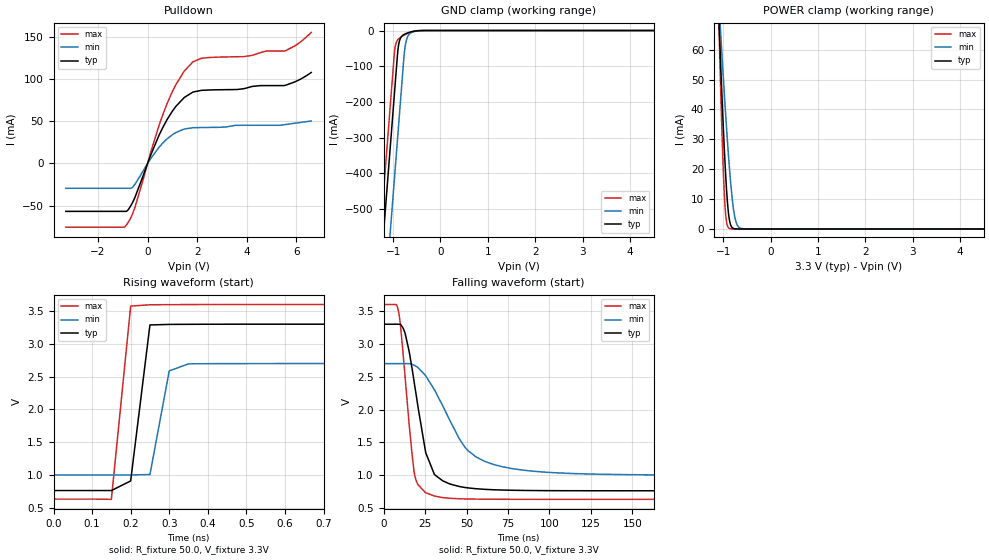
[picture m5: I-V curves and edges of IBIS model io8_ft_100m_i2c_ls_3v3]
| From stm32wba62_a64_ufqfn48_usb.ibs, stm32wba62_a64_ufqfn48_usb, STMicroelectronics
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[Model]   io8_ft_100m_i2c_ls_3v3
Model_type I/O_open_drain
Polarity   Non-Inverting
Enable   Active-Low
| CAP_THRESHOLD on pad IOFT is "UDTCAPC" :
| Rising=30.0% of vddiom   Falling=70.0% of vddiom
| C_comp min and max val. don't necessarily correlate with the min and max pvt
| but are the smallest and greatest pad capacitance found.
| var   typ   min   max
C_comp   3.81294pF  3.70667pF  3.87011pF
|C_comp_pulldown   3.81294pF  3.70667pF  3.87011pF
Vinl = 1.35V
Vinh = 1.8V
Vmeas = 1.65V   | Reference voltage for timing measurements
Cref  = 50.0pF   | Timing specification test load capacitance value
Rref  = 1.0MOhm   | Timing specification test load resistance value
Vref  = 1.815V   | Timing specification test load voltage
[Model Spec]
| TIME_THRESHOLD on pin ZII2CV11 is "CMOS" :
| Rising=50.0% of vdd   Falling=50.0% of vdd
Vinl 1.29050V 1.08050V 1.37650V
Vinh 1.79850V 1.52050V 1.90250V
| variable   typ   min   max
[Temperature Range] 25.0 140.0 -40.0
| variable   typ   min   max
[Voltage Range] 3.3V 2.7V 3.6V
| variable   typ   min   max
[POWER Clamp Reference] 3.3V 2.7V 3.6V
| variable   typ   min   max
[GND Clamp Reference] 0V 0V 0V
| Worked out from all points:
|   slope of the pulldown table from 0 to 0.495 V, typ, clamps not added: 14 ohm
|   GND clamp passes 1 mA (typ) near -0.51 V on its own axis
|   POWER clamp passes 1 mA (typ) near -0.83 V on its own axis
|   rising waveform, R_fixture 50.0, V_fixture 3.3V: 20-80 % time 32ps typ, 32.3ps min, 30.2ps max; typ from 0.764 V to 3.3 V
|   falling waveform, R_fixture 50.0, V_fixture 3.3V: 20-80 % time 10.5ns typ, 23.4ns min, 6.38ns max; typ from 3.3 V to 0.764 V
[POWER Clamp]
-3.3V     1.123A     753mA      1.645A
-1.09V    69.42mA    75.17mA    67.14mA
-1.08V    65.31mA    72.42mA    61.23mA
-1.06V    57.23mA    66.98mA    49.77mA
-1.01V    38.06mA    53.68mA    24.29mA
-970mV    24.36mA    43.46mA    9.575mA
-930mV    13.06mA    33.74mA    2.352mA
-870mV    3.065mA    20.56mA    165.9uA
-810mV    418.4uA    10.06mA    10.3uA
-760mV    69.41uA    4.321mA    1.009uA
-630mV    611.5nA    197uA      2.727nA
6.6V      0A         0A         0A
[GND Clamp]
-3.3V     -4.134A    -4.372A    -4.018A
-1.59V    -1.227A    -1.465A    -1.111A
-1.25V    -648.9mA   -886.9mA   -533mA
-980mV    -189.9mA   -427.9mA   -74mA
-960mV    -155.9mA   -393.9mA   -48.8mA
-910mV    -70.86mA   -308.9mA   -27.2mA
-880mV    -37.23mA   -257.9mA   -22.76mA
-770mV    -11.28mA   -71.59mA   -12.95mA
-730mV    -8.709mA   -32.74mA   -10.07mA
-630mV    -4.122mA   -6.943mA   -4.354mA
-370mV    -42.68uA   -212.2uA   -13.03uA
6.6V      2.311nA    506.4nA    1.057nA
| variable   typ   min   max
[Pullup Reference] 3.3V 2.7V 3.6V
| variable   typ   min   max
[Pulldown Reference] 0V 0V 0V
[Pulldown]
-3.3V     -56.7mA    -29.42mA   -75.36mA
-860mV    -56.67mA   -29.42mA   -72.94mA
-520mV    -40.69mA   -25.01mA   -52.64mA
460mV     33.25mA    19.09mA    44.92mA
800mV     52.54mA    29.36mA    71.75mA
1.14V     67.41mA    36.49mA    93.2mA
1.48V     77.97mA    40.67mA    109.3mA
1.83V     84.38mA    42.18mA    120.1mA
2.17V     86.37mA    42.45mA    124.3mA
3.88V     88.31mA    45.1mA     126.3mA
5.54V     92.28mA    45.89mA    133mA
6.6V      107.5mA    50.2mA     155mA
[Ramp]
dV/dt_r 1.52155V/251.05207ps 1.01897V/339.24608ps 1.7797V/235.85679ps
dV/dt_f 1.52157V/9.99368ns 1.01885V/23.02642ns 1.77971V/6.34242ns
R_load = 50.0
| Removed startup time: 0s 0s 0s  .
| Removed end time: 1.7ns.
[Rising Waveform]
R_fixture   = 50.0
V_fixture   = 3.3V
V_fixture_min = 2.7V
V_fixture_max = 3.6V
0s        764mV      1.002V     633.8mV
150ps     764mV      1.002V     630.3mV
200ps     910.7mV    1.002V     3.576V
250ps     3.288V     1.008V     3.596V
300ps     3.297V     2.588V     3.598V
350ps     3.298V     2.695V     3.599V
1.7ns     3.3V       2.7V       3.6V
| Removed startup time: 0s 0s 0s  .
| Removed end time: 249.25ns.
[Falling Waveform]
R_fixture   = 50.0
V_fixture   = 3.3V
V_fixture_min = 2.7V
V_fixture_max = 3.6V
0s        3.3V       2.7V       3.6V
8.8ns     3.3V       2.7V       3.514V
10.2ns    3.297V     2.7V       3.266V
13.05ns   3.15V      2.7V       2.46V
18.35ns   2.428V     2.676V     1.059V
25.45ns   1.339V     2.511V     734.5mV
31.15ns   1V         2.276V     680.6mV
49ns      814.2mV    1.427V     640mV
66.15ns   779.7mV    1.165V     635.1mV
249.3ns   764mV      1.002V     633.8mV
